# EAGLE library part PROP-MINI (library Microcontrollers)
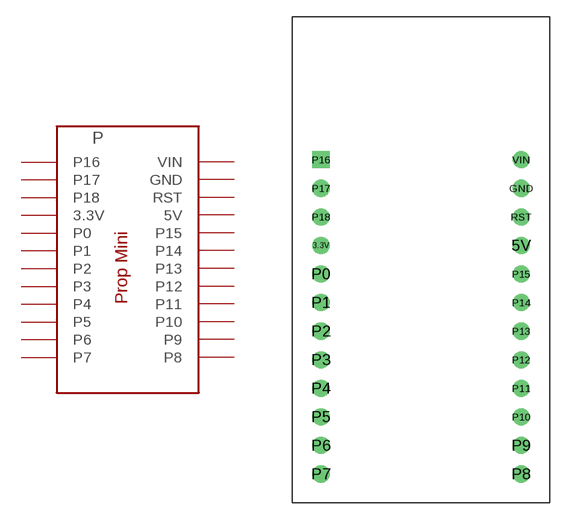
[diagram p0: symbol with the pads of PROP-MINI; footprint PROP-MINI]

Designator prefix P

## PROP-MINI  [PROP-MINI]
3.3V  3.3V
5V  5V
GND  GND
P0  P0
P1  P1
P2  P2
P3  P3
P4  P4
P5  P5
P6  P6
P7  P7
P8  P8
P9  P9
P10  P10
P11  P11
P12  P12
P13  P13
P14  P14
P15  P15
P16  P16
P17  P17
P18  P18
RST  RST
VIN  VIN

## Footprint PROP-MINI (pad centres in mm)
drill 1.016: 3.3V -8.89,6.35; 5V 8.89,6.35; GND 8.89,11.43; P0 -8.89,3.81; P1 -8.89,1.27; P2 -8.89,-1.27; P3 -8.89,-3.81; P4 -8.89,-6.35; P5 -8.89,-8.89; P6 -8.89,-11.43; P7 -8.89,-13.97; P8 8.89,-13.97; P9 8.89,-11.43; P10 8.89,-8.89; P11 8.89,-6.35; P12 8.89,-3.81; P13 8.89,-1.27; P14 8.89,1.27; P15 8.89,3.81; P17 -8.89,11.43; P18 -8.89,8.89; RST 8.89,8.89; VIN 8.89,13.97
drill 1.016 square: P16 -8.89,13.97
